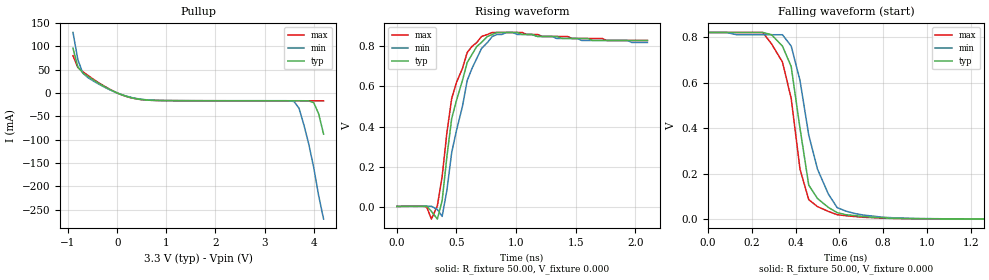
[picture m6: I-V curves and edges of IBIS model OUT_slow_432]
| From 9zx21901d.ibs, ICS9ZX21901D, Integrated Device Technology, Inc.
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|   Model OUT_slow_432
[Model]   OUT_slow_432
Model_type   Open_source
Polarity   Non-Inverting
Enable   Active-High
Vmeas =  0.350V
Cref =   2.00pF
Rref =  70.000
Vref =   0.350V
C_comp   3.40pF   2.85pF   3.95pF
[Temperature Range]   27.00   70.00   0.000
[Voltage Range]   3.30V   3.00V   3.60V
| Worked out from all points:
|   slope of the pullup table from 0 to 0.495 V, typ, clamps not added: 35.4 ohm
|   rising waveform, R_fixture 50.00, V_fixture 0.000: 20-80 % time 160ps typ, 170ps min, 149ps max; typ from 0.001 V to 0.83 V
|   falling waveform, R_fixture 50.00, V_fixture 0.000: 20-80 % time 75.6ps typ, 118ps min, 88.1ps max; typ from 0.82 V to 0.001 V
[Pullup]
| voltage   I(typ)   I(min)   I(max)
|  -3.30   2.07A   2.09A   2.05A
  |-3.10   1.90A   1.92A   1.88A
  |-2.90   1.73A   1.75A   1.71A
  |-2.70   1.56A   1.58A   1.54A
  |-2.50   1.39A   1.42A   1.37A
  |-2.30   1.22A   1.25A   1.20A
  |-2.10   1.05A   1.08A   1.03A
  |-1.90   0.89A   0.92A   0.87A
  |-1.70   0.72A   0.75A   0.70A
  |-1.50   0.56A   0.59A   0.53A
  |-1.00   0.16A   0.20A   0.14A
-900mV    96.29mA    130mA      80.29mA
-800mV    55.8mA     71.37mA    54.73mA
-700mV    43.51mA    42.75mA    45.88mA
-300mV    16.29mA    15.02mA    17.28mA
200mV     -7.39mA    -6.93mA    -7.73mA
800mV     -15.74mA   -15.59mA   -15.8mA
3.6V      -16.37mA   -18.13mA   -16.43mA
3.7V      -16.38mA   -32.38mA   -16.44mA
3.9V      -16.78mA   -110mA     -16.44mA
4V        -20.49mA   -160mA     -16.44mA
4.1V      -44.46mA   -220mA     -16.45mA
4.2V      -87.94mA   -270mA     -16.64mA
  | 4.30   -0.14A   -0.32A   -18.12mA
   |4.50   -0.25A   -0.43A   -71.28mA
   |4.70   -0.36A   -0.54A   -0.17A
   |4.90   -0.47A   -0.65A   -0.29A
   |5.10   -0.58A   -0.77A   -0.40A
   |5.30   -0.70A   -0.88A   -0.51A
   |5.50   -0.81A   -0.99A   -0.63A
   |5.70   -0.93A   -1.10A   -0.75A
   |5.90   -1.04A   -1.21A   -0.86A
   |6.10   -1.16A   -1.33A   -0.98A
   |6.60   -1.45A   -1.61A   -1.27A
[Ramp]
| variable   typ   min   max
dV/dt_r   0.49/0.16n   0.49/0.17n   0.50/0.16n
dV/dt_f   0.49/97.37p   0.49/0.11n   0.49/89.64p
R_load = 50.00
[Rising Waveform]
R_fixture = 50.00
V_fixture = 0.000
V_fixture_min = 0.000
V_fixture_max = 0.000
| time   V(typ)   V(min)   V(max)
0s        720uV      630uV      790uV
250ps     2.49mV     1.59mV     -1.59mV
290ps     -23.92mV   1.55mV     -62.32mV
340ps     -62.48mV   -14.62mV   3.75mV
380ps     29.41mV    -49.2mV    150mV
460ps     440mV      270mV      540mV
590ps     720mV      630mV      770mV
710ps     820mV      790mV      850mV
920ps     870mV      870mV      870mV
2.1ns     830mV      820mV      830mV
[Falling Waveform]
R_fixture = 50.00
V_fixture = 0.000
V_fixture_min = 0.000
V_fixture_max = 0.000
| time   V(typ)   V(min)   V(max)
0s        820mV      820mV      820mV
250ps     820mV      810mV      820mV
340ps     760mV      810mV      690mV
380ps     670mV      760mV      530mV
420ps     400mV      610mV      220mV
460ps     150mV      370mV      85.93mV
550ps     51.59mV    110mV      34.1mV
590ps     28.81mV    50.95mV    19.74mV
800ps     5.88mV     8.57mV     4.36mV
2.1ns     730uV      640uV      790uV
